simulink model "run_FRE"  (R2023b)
settings: configuration reference "FRE_simulation_config" (kept in a data dictionary, not in this file)
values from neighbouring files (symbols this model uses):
  FRE_time_step = 0.005
                
                    
                        1
                        Auto
                        
                        
                        -1.0
                        0
                        Simulink
                        Parameter
                        Default    [run_FRE_data.sldd]
  frequency_vector = logspace(log10(min_estimation_frequency), log10(max_estimation_frequency), estimation_frequency_point_num)
                                
                            
                        
                    
                
                
                    
                        1
                        Auto
                        
                        
                        -    [run_FRE_data.sldd]
undefined symbols (not defined in the file or in its folder): action, control, perturbation
libraries: slctrl_fre x1, SignalEditorBlockLib x1

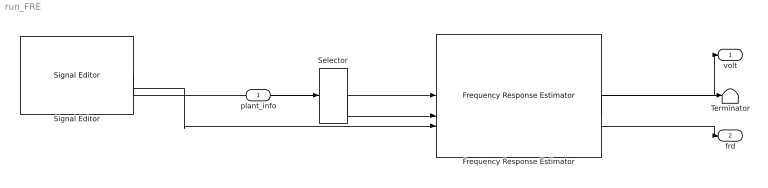
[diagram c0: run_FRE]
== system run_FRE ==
  plant_info : Inport  OutDataTypeStr=single  PortDimensions=4
  Frequency Response Estimator : slctrl_fre/Frequency Response Estimator  DiscreteTs=FRE_time_step  OutputMode=control action + perturbation  BlockDataType=single  SineSource=Block parameters  Frequencies=[frequency_vector]  FreqUnits=Hz  Amplitudes=FRE_amplitude  NumOfFreq=3  ExperimentMode=PRBS  NumOfSetPeriod=2  NumOfEstPeriod=4  NumOfSlowestPeriod=3  NumOfPRBSPeriod=1  UseAutogenNumOfPRBSPeriod=on  PRBSSignalOrder=12  UseAutogenPRBSSignalOrder=on  EstimationMode=Online  UseBodePlot=off  BaselinePlant=[]  PlotRefreshFactor=100  UseExternalTs=off  BodePlotChoice=VariantNull  ExperimentChoice=VariantPRBS  OutputChoice=VariantCandD  CompiledTsChoice=InternalTs
  Selector : Selector  InputPortWidth=4  IndexOptions=Index vector (dialog)  Indices=[3]  OutputSizes=1
  Signal Editor : SignalEditorBlockLib/Signal Editor  FileName=FRE_input_data.mat  ActiveScenario=FRE_operation  ActiveSignal=u  IsBus=off  OutputBusObjectStr=Bus: BusObject  SampleTime=FRE_time_step  Interpolate=off  ZeroCross=off  OutputAfterFinalValue=Holding final value  Unit=inherit  PreserveSignalName=on  ApplySigPropsToAllScenarios=on  ApplySigPropsToAllSignals=on
  Terminator : Terminator
  volt : Outport  PortDimensions=1
  frd : Outport  Port=2
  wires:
  Signal Editor/1 -> Frequency Response Estimator/1
  plant_info/1 -> Selector/1
  Signal Editor/2 -> Frequency Response Estimator/3
  Selector/1 -> Frequency Response Estimator/2
  Frequency Response Estimator/1 -> volt/1
  Frequency Response Estimator/3 -> frd/1
  Frequency Response Estimator/2 -> Terminator/1
